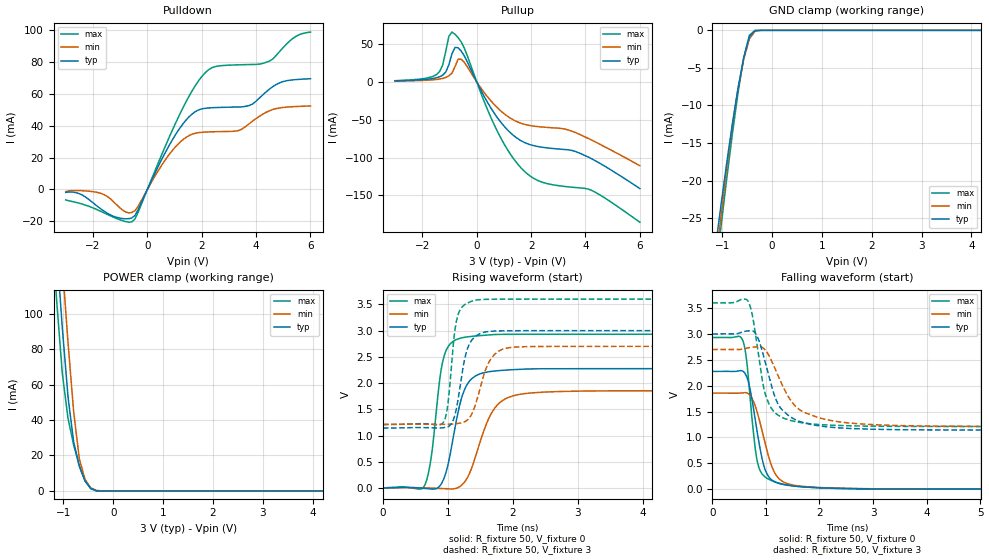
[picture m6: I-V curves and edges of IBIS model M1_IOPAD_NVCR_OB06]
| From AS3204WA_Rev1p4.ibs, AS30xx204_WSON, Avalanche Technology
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[Model] M1_IOPAD_NVCR_OB06
Model_type I/O
Enable   Active-High
Vinl  =  0.9
Vinh  =  2.1
Vmeas =  1.5
Cref  =  30e-12
| Capacitance  typ   min   max
C_comp   3.872127e-12   3.590660e-12   4.176448e-12
| Variables   typ   min   max
[GND Clamp Reference]   0   0   0
[POWER Clamp Reference]   3   2.7   3.6
[Pulldown Reference]   0   0   0
[Pullup Reference]   3   2.7   3.6
[Temperature Range]   25   105   -40
[Voltage Range]   3   2.7   3.6
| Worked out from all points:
|   slope of the pulldown table from 0 to 0.45 V, typ, clamps not added: 27.9 ohm
|   slope of the pullup table from 0 to 0.45 V, typ, clamps not added: 14.9 ohm
|   GND clamp passes 1 mA (typ) near -0.46 V on its own axis
|   POWER clamp passes 1 mA (typ) near -0.42 V on its own axis
|   falling waveform, R_fixture 50, V_fixture 0: 20-80 % time 236ps typ, 300ps min, 174ps max; typ from 2.28 V to 0 V
|   falling waveform, R_fixture 50, V_fixture 3: 20-80 % time 382ps typ, 533ps min, 253ps max; typ from 3 V to 1.14 V
|   rising waveform, R_fixture 50, V_fixture 0: 20-80 % time 235ps typ, 337ps min, 166ps max; typ from 0 V to 2.28 V
|   rising waveform, R_fixture 50, V_fixture 3: 20-80 % time 164ps typ, 233ps min, 114ps max; typ from 1.14 V to 3 V
[GND Clamp]
| Voltage   I(typ)   I(min)   I(max)
-3V       -145.9mA   -151.9mA   -144.2mA
-1.138V   -29.07mA   -31.55mA   -32.68mA
-1.024V   -23.24mA   -24.83mA   -26.15mA
-910.3mV  -17.69mA   -18.46mA   -19.83mA
-796.6mV  -12.47mA   -12.67mA   -13.82mA
-682.8mV  -7.718mA   -7.754mA   -8.316mA
-569mV    -3.663mA   -3.867mA   -3.675mA
-455.2mV  -839.2uA   -1.152mA   -666.1uA
-341.4mV  -35.63uA   -111.1uA   -11.17uA
-113.8mV  -8.642nA   -188.3nA   -1.888nA
6V        0A         0A         0A
[POWER Clamp]
| Voltage   I(typ)   I(min)   I(max)
-3V       949.8mA    984.2mA    923.5mA
-1.252V   183.6mA    221.4mA    154mA
-1.138V   136.7mA    174.2mA    107.6mA
-1.024V   92.09mA    128.1mA    66.35mA
-910.3mV  53.33mA    83.97mA    41.06mA
-796.6mV  27.72mA    44.75mA    25.94mA
-682.8mV  13.75mA    18.06mA    14.29mA
-569mV    5.664mA    6.605mA    5.738mA
-455.2mV  1.446mA    1.789mA    1.305mA
-341.4mV  77.09uA    287.6uA    62.73uA
-227.6mV  1.148uA    12.92uA    332nA
6V        0A         0A         0A
[Pulldown]
| Voltage   I(typ)   I(min)   I(max)
-3V       -1.818mA   -1.307mA   -6.547mA
-2.39V    -3.494mA   -774.4uA   -9.164mA
-1.707V   -12.21mA   -2.448mA   -13.76mA
-569mV    -17.8mA    -14.41mA   -20.26mA
1.034V    34.32mA    26.75mA    41.44mA
1.552V    45.85mA    33.95mA    59.04mA
2.069V    50.76mA    35.95mA    72.13mA
2.483V    51.35mA    36.22mA    76.98mA
3.745V    52.65mA    41.22mA    78.33mA
4.49V     62.91mA    49.37mA    80.49mA
5.359V    68.75mA    51.92mA    94.81mA
6V        69.43mA    52.36mA    98.69mA
[Pullup]
| Voltage   I(typ)   I(min)   I(max)
-3V       1.233mA    920.2uA    1.446mA
-1.479V   5.373mA    3.102mA    9.525mA
-1.252V   8.683mA    4.453mA    22.01mA
-1.138V   12.76mA    5.671mA    40.18mA
-910.3mV  37mA       11.54mA    65.62mA
-796.6mV  45.31mA    20.09mA    62.75mA
-569mV    40.45mA    29.77mA    52.57mA
724.1mV   -45.54mA   -33mA      -62.73mA
1.655V    -78.26mA   -55.05mA   -114.6mA
2.379V    -86.23mA   -59.61mA   -132.2mA
3.745V    -93.6mA    -68.79mA   -139.9mA
6V        -141mA     -110.8mA   -185.3mA
[Ramp]
dV/dt_r   1.36569/0.235041n  1.1138/0.336884n  1.75879/0.166379n
dV/dt_f   1.11466/0.381872n  0.893766/0.532893n  1.43365/0.253146n
R_load = 50
[Falling Waveform]
R_fixture = 50
V_fixture = 0
V_fixture_min = 0
V_fixture_max = 0
| Time   V(typ)   V(min)   V(max)
0s        2.276V     1.856V     2.931V
554.1ps   2.289V     1.862V     2.908V
626.6ps   2.209V     1.866V     2.606V
693ps     1.996V     1.827V     1.931V
801.9ps   1.342V     1.608V     787.8mV
880ps     855.4mV    1.331V     390.8mV
998.2ps   347.1mV    839.4mV    227.1mV
1.171ns   139.8mV    306.1mV    139.9mV
1.56ns    56.31mV    69.92mV    56.31mV
21.88ns   748.7nV    811.1nV    11.74uV
[Falling Waveform]
R_fixture = 50
V_fixture = 3
V_fixture_min = 2.7
V_fixture_max = 3.6
| Time   V(typ)   V(min)   V(max)
0s        3V         2.7V       3.6V
654.8ps   3.059V     2.73V      3.653V
737.2ps   3.06V      2.743V     3.421V
841.1ps   2.951V     2.75V      2.755V
956.6ps   2.58V      2.723V     1.976V
1.062ns   2.159V     2.574V     1.639V
1.276ns   1.567V     2.082V     1.4V
1.799ns   1.26V      1.453V     1.267V
4.127ns   1.145V     1.218V     1.212V
21.88ns   1.142V     1.21V      1.211V
[Rising Waveform]
R_fixture = 50
V_fixture = 0
V_fixture_min = 0
V_fixture_max = 0
| Time   V(typ)   V(min)   V(max)
0s        455.7nV    464.4nV    11.7uV
646.1ps   -3.297mV   7.44mV     61.69mV
745.3ps   -14.7mV    3.031mV    600.1mV
875.5ps   41.5mV     -4.152mV   2.072V
944.4ps   202.1mV    -8.401mV   2.525V
1.189ns   1.614V     33.98mV    2.854V
1.342ns   2.05V      305.3mV    2.888V
1.766ns   2.237V     1.59V      2.927V
2.391ns   2.273V     1.824V     2.93V
21.88ns   2.276V     1.856V     2.931V
[Rising Waveform]
R_fixture = 50
V_fixture = 3
V_fixture_min = 2.7
V_fixture_max = 3.6
| Time   V(typ)   V(min)   V(max)
0s        1.142V     1.21V      1.211V
928.5ps   1.15V      1.215V     1.248V
995.4ps   1.168V     1.216V     1.553V
1.099ns   1.352V     1.223V     2.914V
1.158ns   1.688V     1.232V     3.303V
1.29ns    2.611V     1.287V     3.517V
1.484ns   2.937V     1.847V     3.588V
1.704ns   2.99V      2.527V     3.597V
2.119ns   2.998V     2.692V     3.599V
21.88ns   3V         2.7V       3.6V
